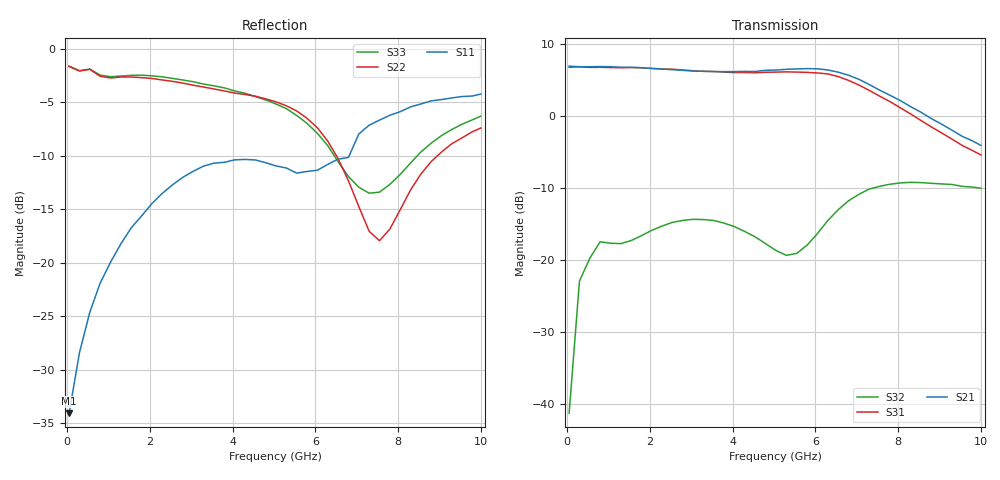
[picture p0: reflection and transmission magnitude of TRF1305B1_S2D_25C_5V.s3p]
! Created Tue Jun 24 15:01:08 2025
# hz S ma R 50
! 3 Port Network Data from SP1.SP block
! PORT[1] = INP
! PORT[2] = OUTM
! PORT[3] = OUTP
! freq  magS11  angS11  magS12  angS12  magS13  angS13
!  magS21  angS21
!  magS22  angS22  magS23  angS23
!  magS31  angS31  magS32  angS32
!  magS33  angS33
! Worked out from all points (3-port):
!   41 points, 50 MHz to 10 GHz, reference 50 ohm
!   strongest paths, dB at 50 MHz, 2.55 GHz, 5.05 GHz, 7.55 GHz, 10 GHz:
!     S21: 6.9, 6.4, 6.4, 3.6, -4.1
!     S31: 6.8, 6.5, 6.1, 2.7, -5.4
!     S32: -41.3, -14.8, -18.7, -9.8, -10.1
!   lowest |S11| = -34.0 dB at 50 MHz (marker M1), VSWR 1.04, Z = 48.1 - j0.5 ohm
!   |S11| at or under -10 dB: start of sweep to 6.816 GHz
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5e7  0.01984 -164.8  0.0008615 -51.0  0.003061 140.3
     2.213 178.1  0.8285 178.6  0.008164 123.3
     2.176 -2.0  0.008584 119.9  0.831 178.2
3e8  0.03809 -136.7  0.01654 47.8  0.01281 61.8
     2.193 168.4  0.7887 171.0  0.06898 55.3
     2.186 -11.1  0.07108 53.0  0.7918 171.2
1.55e9  0.1459 -148.8  0.04635 24.9  0.0314 15.1
        2.175 120.8  0.7395 149.2  0.136 24.8
        2.166 -56.9  0.136 22.8  0.7532 149.7
2.3e9  0.2114 -169.1  0.06121 9.3  0.04008 -4.6
       2.112 92.4  0.7164 133.9  0.1771 13.3
       2.117 -85.1  0.1716 11.1  0.7409 133.9
3.8e9  0.2953 144.9  0.08526 -29.0  0.05827 -61.5
       2.027 38.8  0.6365 106.3  0.1788 -32.1
       2.011 -139.9  0.1795 -34.7  0.6579 105.5
5.05e9  0.2841 116.4  0.09427 -57.9  0.05839 -116.5
        2.08 -8.4  0.5661 81.5  0.09734 -99.3
        2.012 172.2  0.116 -104.1  0.553 82.3
5.8e9  0.2677 112.8  0.1051 -75.5  0.05348 -150.1
       2.128 -40.8  0.474 62.8  0.0963 168.2
       2.004 139.4  0.1264 175.2  0.4489 67.5
6.55e9  0.3056 113.4  0.1136 -95.5  0.03877 175.4
        2.011 -77.6  0.3072 45.6  0.1898 105.9
        1.875 101.6  0.2226 112.8  0.2975 61.2
7.8e9  0.4901 94.4  0.1066 -134.5  0.02321 133.4
       1.39 -133.7  0.144 98.6  0.3061 50.3
       1.257 43.8  0.3348 50.6  0.2329 98.7
1e10  0.6158 49.0  0.07668 172.1  0.01103 76.0
      0.6226 156.8  0.4272 94.2  0.3217 -0.6
      0.5347 -28.0  0.3139 -3.2  0.4857 93.8
